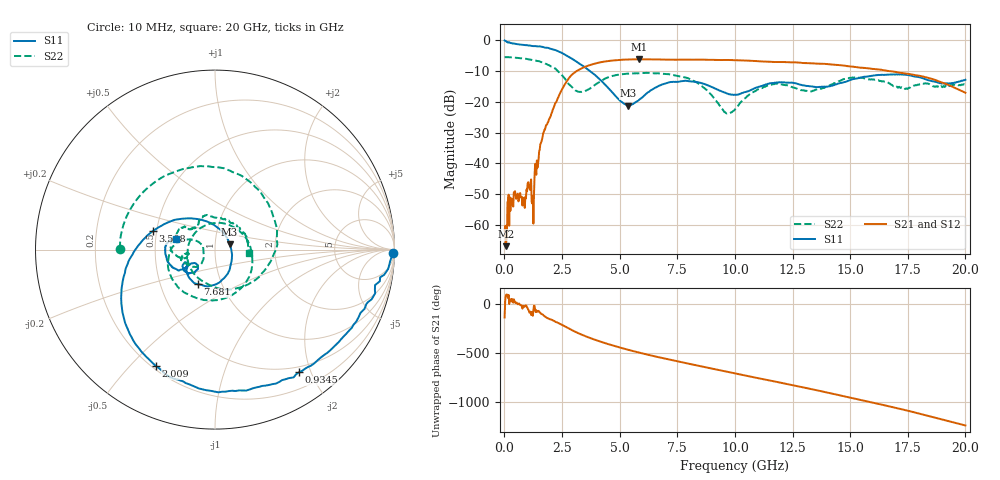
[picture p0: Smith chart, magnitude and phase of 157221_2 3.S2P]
!  2-Port S-parameters saved by WinCal
! VAR MeasName=S-Parameters (CALIBRATED_DATA) read from VNA (N5242A)
! VAR MeasDate=2015-5-26 16:47:27
! VAR NAME=157221_2 3
! VAR FILENAME=157221_2 3.S2P
! VAR DATE=2015-5-26 16:47:27
! VAR PHYS_PORTS=1,2
# Hz S DB R 50
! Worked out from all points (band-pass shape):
!   801 points, 10 MHz to 20 GHz, reference 50 ohm
!   highest |S21| = -6.20 dB at 5.857 GHz (marker M1); lowest = -66.9 dB at 59.98 MHz (marker M2)
!   |S21| within 3 dB of the highest: 3.332 GHz to 15.86 GHz (12.52 GHz wide, 131 % of centre)
!   lowest |S11| = -21.2 dB at 5.382 GHz (marker M3), VSWR 1.19, Z = 58.7 + j3.62 ohm
!   |S11| at or under -10 dB: 3.716 GHz to end of sweep
!   |S22| runs from -23.8 to -5.5 dB; largest |S21 - S12| = 0.0097
!   S11 on the Smith chart (normalised r, x): 10 MHz: 37, -82; 934.5 MHz: 0.42, -1.82; 2.009 GHz: 0.22, -0.59; 3.508 GHz: 0.48, +0.11; 7.681 GHz: 0.77, -0.31; 20 GHz: 0.64, +0.08
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1e7  -0.08 -1.2  -61.88 -141.0  -70.37 -170.1  -5.53 179.5
5.9975e7  -0.26 -6.4  -66.93 81.5  -67.64 75.1  -5.52 176.6
2.348875e8  -0.76 -17.6  -51.00 27.5  -50.80 27.0  -5.54 166.7
9.345375e8  -1.64 -55.7  -51.44 -18.1  -51.32 -19.1  -6.05 125.5
1.284362e9  -1.93 -74.7  -50.12 -20.7  -50.17 -20.2  -6.50 101.9
1.6092e9  -2.10 -93.4  -32.92 -105.9  -32.88 -106.2  -7.11 74.9
2.009e9  -2.77 -117.0  -24.66 -160.2  -24.62 -160.5  -8.45 32.3
2.633688e9  -4.72 -154.1  -14.21 128.0  -14.19 127.7  -12.53 -71.0
3.358325e9  -8.12 170.0  -9.10 44.2  -9.09 43.8  -16.80 116.4
3.50825e9  -8.87 163.2  -8.62 29.7  -8.61 29.4  -16.49 85.4
4.257875e9  -13.60 124.4  -7.04 -32.8  -7.05 -33.1  -12.95 -23.6
5.382312e9  -21.22 20.6  -6.24 -109.6  -6.25 -109.7  -10.85 -101.1
5.857075e9  -19.33 -29.9  -6.20 -138.0  -6.23 -138.2  -10.73 -120.4
6.681662e9  -14.91 -79.8  -6.26 176.4  -6.24 176.3  -10.77 -145.5
7.681162e9  -13.32 -116.6  -6.33 125.6  -6.31 125.3  -11.86 -175.2
1.0005e10  -17.69 -138.9  -6.49 11.6  -6.49 11.1  -22.52 -146.2
1.177911e10  -13.82 -142.5  -7.08 -73.1  -7.02 -74.0  -14.11 -162.5
1.335332e10  -15.02 -155.7  -7.52 -150.1  -7.48 -150.5  -16.54 -170.5
1.52024e10  -12.54 -150.6  -8.67 115.3  -8.59 114.9  -12.10 174.7
1.667666e10  -11.19 -173.8  -10.01 37.3  -10.00 37.0  -13.97 143.4
1.837581e10  -12.98 164.3  -12.22 -59.2  -12.19 -60.4  -14.10 102.7
2e10  -12.86 165.1  -17.06 -157.2  -17.10 -158.6  -14.31 -5.5
